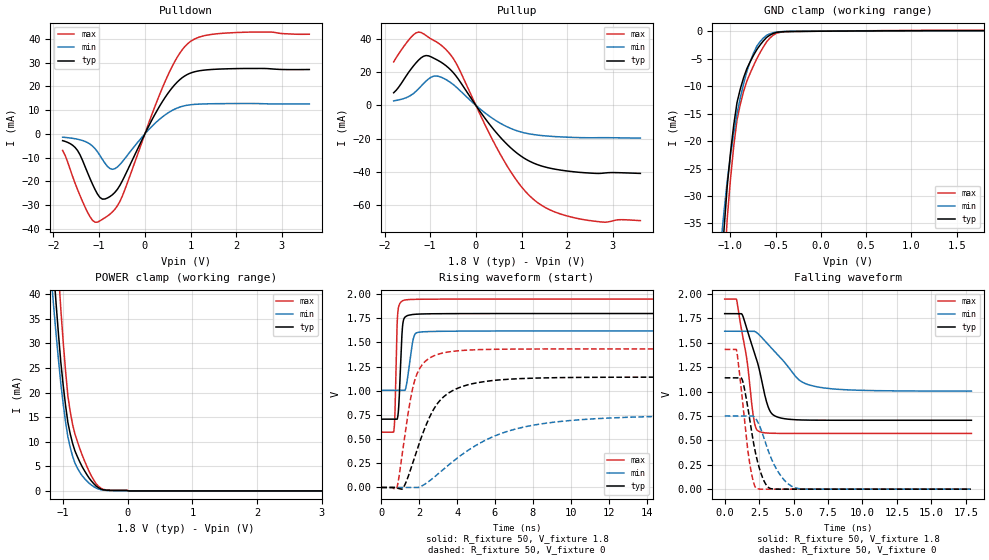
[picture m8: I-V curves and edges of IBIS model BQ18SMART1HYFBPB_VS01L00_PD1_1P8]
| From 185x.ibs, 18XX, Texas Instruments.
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|   Model Cell BQ18SMART1HYFBPB_VS01L00_PD1_1P8
|BQ18SMART1HYFBPB_VS01L00_PD1_1P8
[Model]   BQ18SMART1HYFBPB_VS01L00_PD1_1P8
Model_type   I/O
Polarity   Non-Inverting
Enable   Active-Low
Vinl =  0.63
Vinh =  1.17
Cref =  15pF
Rref =  100.0000M
Vref =  0V
Vmeas =  0.9
C_comp   0.9029199p   0.7983694p   1.014934p
[Model Spec]
Vinl   0.63   0.567   0.6825
Vinh   1.17   1.053   1.2675
[Temperature Range]   25   125   -40
[Voltage Range]   1.8   1.62   1.95
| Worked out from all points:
|   slope of the pulldown table from 0 to 0.27 V, typ, clamps not added: 27.2 ohm
|   slope of the pullup table from 0 to 0.27 V, typ, clamps not added: 26 ohm
|   GND clamp passes 1 mA (typ) near -0.59 V on its own axis
|   POWER clamp passes 1 mA (typ) near -0.49 V on its own axis
|   rising waveform, R_fixture 50, V_fixture 1.8: 20-80 % time 145ps typ, 263ps min, 101ps max; typ from 0.706 V to 1.8 V
|   rising waveform, R_fixture 50, V_fixture 0: 20-80 % time 1.54ns typ, 3.83ns min, 767ps max; typ from 0 V to 1.14 V
|   falling waveform, R_fixture 50, V_fixture 1.8: 20-80 % time 1.24ns typ, 2.27ns min, 814ps max; typ from 1.8 V to 0.706 V
|   falling waveform, R_fixture 50, V_fixture 0: 20-80 % time 900ps typ, 1.34ns min, 683ps max; typ from 1.14 V to 0 V
| Nom Voltages:
|   BIASFET=1.8, VBBNW=1.1, VDD=1.1, VDDS=1.8, VSS=0, VSSS=0
| Min Voltages:
|   BIASFET=1.62, VBBNW=0.99, VDD=0.99, VDDS=1.62, VSS=0, VSSS=0
| Max Voltages:
|   BIASFET=1.95, VBBNW=1.21, VDD=1.21, VDDS=1.95, VSS=0, VSSS=0
[POWER_clamp]
|   voltage   I(typ)   I(min)   I(max)
-1.8V     196.9mA    157.5mA    250.4mA
-1.182V   51.67mA    43mA       68.61mA
-1.145V   44.45mA    37.16mA    60.1mA
-1.109V   37.9mA     31.74mA    52.07mA
-1.073V   31.79mA    26.6mA     44.33mA
-1.036V   26.12mA    21.74mA    36.87mA
-963.6mV  17.39mA    14.07mA    24.42mA
-927.3mV  13.91mA    10.96mA    19.29mA
-854.5mV  9.657mA    7.054mA    13.5mA
-709.1mV  4.995mA    3.131mA    7.393mA
-490.9mV  991uA      585.4uA    1.466mA
3.6V      0A         0A         0A
[Pulldown]
|   voltage   I(typ)   I(min)   I(max)
-1.8V     -2.835mA   -1.376mA   -6.938mA
-1.473V   -6.994mA   -2.229mA   -23.44mA
-1.2V     -18.79mA   -4.282mA   -34.89mA
-1.036V   -25.34mA   -7.531mA   -37.14mA
-872.7mV  -27.39mA   -12.36mA   -35.28mA
-654.5mV  -24.59mA   -14.63mA   -31.68mA
-490.9mV  -19.69mA   -11.65mA   -26.08mA
381.8mV   13.54mA    7.116mA    19.32mA
654.5mV   20.72mA    10.44mA    30.47mA
927.3mV   25mA       12.07mA    37.79mA
1.636V    27.3mA     12.74mA    42.26mA
3.6V      27.12mA    12.64mA    41.97mA
[Pullup]
|   voltage   I(typ)   I(min)   I(max)
-1.8V     7.614mA    2.74mA     26.22mA
-1.527V   17.69mA    4.626mA    37.43mA
-1.309V   25.69mA    8.541mA    43.72mA
-1.036V   29.87mA    15.94mA    41.05mA
-818.2mV  26.95mA    17.52mA    37.49mA
-490.9mV  19.61mA    12.45mA    28.08mA
545.5mV   -19.54mA   -10.94mA   -30.03mA
927.3mV   -29.38mA   -15.56mA   -46.58mA
1.255V    -34.7mA    -17.56mA   -56.51mA
1.691V    -38.25mA   -18.74mA   -63.85mA
2.291V    -40.42mA   -19.45mA   -68.55mA
3.6V      -41.01mA   -19.75mA   -69.5mA
[GND_clamp]
|   voltage   I(typ)   I(min)   I(max)
-1.8V     -274mA     -200.4mA   -365.5mA
-1.109V   -45.41mA   -39.33mA   -55.91mA
-1.073V   -36.49mA   -33.11mA   -44.46mA
-1.036V   -28.34mA   -27.37mA   -34.29mA
-1V       -22.19mA   -22.71mA   -27mA
-927.3mV  -12.97mA   -14.93mA   -16.12mA
-854.5mV  -8.452mA   -9.555mA   -10.93mA
-781.8mV  -5.549mA   -5.539mA   -7.634mA
-709.1mV  -3.363mA   -2.741mA   -5.028mA
-600mV    -1.121mA   -737.1uA   -1.924mA
-381.8mV  -62.21uA   -38.42uA   -93.33uA
1.8V      98.66uA    51.35uA    168.2uA
[Ramp]
| variable   typ   min   max
dV/dt_f 0.65730853/1.2434438n 0.37033832/2.2810307n 0.82835907/0.81703934n
dV/dt_r 0.69503053/1.548738n  0.45750728/3.9662333n 0.86864253/0.77004361n
R_load = 50
[Rising Waveform]
R_fixture = 50
V_fixture = 1.8
V_fixture_min = 1.62
V_fixture_max = 1.95
|   time   V(typ)   V(min)   V(max)
0s        705.9mV    1.004V     572mV
660.6ps   705.9mV    1.004V     585.2mV
717.8ps   705.9mV    1.004V     760.3mV
815.7ps   705.9mV    1.004V     1.571V
862ps     725.1mV    1.004V     1.79V
1.156ns   1.718V     1.004V     1.933V
1.325ns   1.772V     1.058V     1.941V
1.689ns   1.789V     1.538V     1.945V
1.954ns   1.793V     1.604V     1.946V
17.91ns   1.798V     1.619V     1.948V
[Rising Waveform]
R_fixture = 50
V_fixture = 0
V_fixture_min = 0
V_fixture_max = 0
|   time   V(typ)   V(min)   V(max)
0s        0V         0V         0V
811.6ps   -2.373mV   0V         -9.826mV
1.172ns   0V         0V         446.1mV
1.496ns   156.9mV    0V         863.9mV
1.743ns   304.9mV    0V         1.094V
2.114ns   518.8mV    13.7mV     1.257V
2.788ns   816.5mV    106mV      1.362V
4.277ns   1.044V     343mV      1.417V
7.5ns     1.127V     623.9mV    1.431V
17.87ns   1.141V     741.3mV    1.432V
[Falling Waveform]
R_fixture = 50
V_fixture = 1.8
V_fixture_min = 1.62
V_fixture_max = 1.95
|   time   V(typ)   V(min)   V(max)
0s        1.798V     1.618V     1.947V
872.4ps   1.798V     1.618V     1.936V
1.616ns   1.638V     1.618V     1.322V
2.099ns   1.426V     1.618V     728.7mV
2.428ns   1.274V     1.592V     596.7mV
3.202ns   826.5mV    1.475V     573.9mV
4.002ns   731.3mV    1.355V     571.4mV
5.435ns   709.3mV    1.115V     571mV
6.785ns   706.4mV    1.046V     571mV
17.91ns   705.8mV    1.004V     571mV
[Falling Waveform]
R_fixture = 50
V_fixture = 0
V_fixture_min = 0
V_fixture_max = 0
|   time   V(typ)   V(min)   V(max)
0s        1.141V     750mV      1.431V
861.3ps   1.141V     750mV      1.423V
1.282ns   1.117V     750mV      920.4mV
1.736ns   787.8mV    750mV      339.3mV
2.039ns   518.2mV    749.2mV    100.3mV
2.305ns   328.1mV    711.9mV    7.003mV
3.165ns   19.1mV     391.6mV    0V
4.136ns   0V         125.1mV    0V
5.147ns   0V         12.55mV    0V
17.87ns   0V         0V         0V
